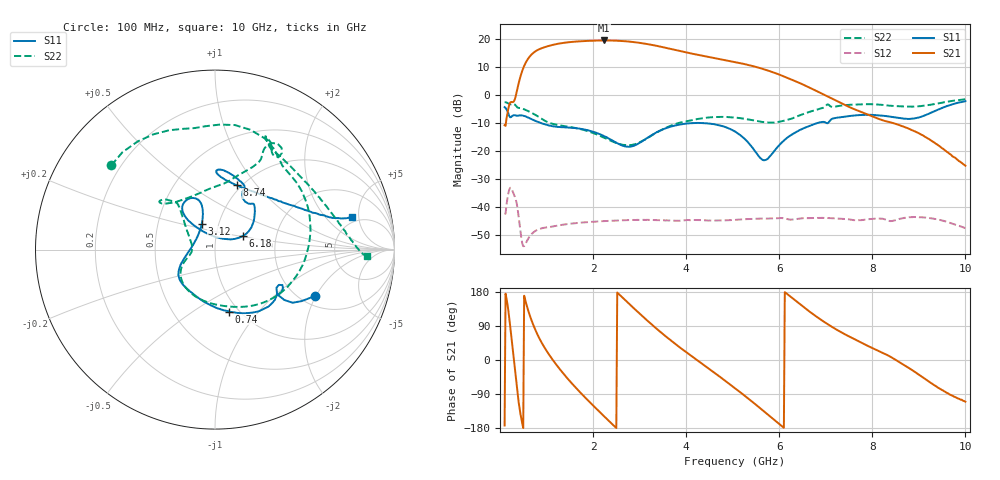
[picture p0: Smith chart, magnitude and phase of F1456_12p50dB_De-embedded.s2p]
! Integrated Device Technology
! Corporate Headquarters
! 6024 Silver Creek Valley Road
! San Jose, CA 95138  USA
! Phone:  1-408-284-8200
! Toll Free:  1-800-223-1366
! Webpage:  http://www.idt.com/
! Timing and RF Division
! 515 Groton Road, Suite 102
! Westford, MA 01886-6024
! Device:  F1456
! Description: 6-bit 0.5 dB Transmit Variable Gain Amplifier
! Frequency:  2100.0 -  2950.00 MHz
! Package:  6x6 mm Thin QFN Plastic Package: 28 pin
! State:  25
! Atten State:  12.5 dB
! Voltage:  +5.00 Volts
! Current:  216.995 mA
! Data:  The device was measured on a the F1455 evaluation board which has
!  individual transmission lines to the RF pins.  Data was collected
!  using a calibrated network analyzer.  The evaluation board was
!  de-embedded using a TRL calibration technique.
!  The reference plane is the edge of the package pin.
!  Pin  1 = CSb
!  Pin  2 = DATA
!  Pin  3 = CLK
!  Pin  4 = RSET
!  Pin  5 = GND
!  Pin  6 = RFIN  = Port 1
!  Pin  7 = GND
!  Pin  8 = NC
!  Pin  9 = NC
!  Pin 10 = NC
!  Pin 11 = NC
!  Pin 12 = NC
!  Pin 13 = NC
!  Pin 14 = /STBY
!  Pin 15 = GND
!  Pin 16 = RFOUT  = Port 2
!  Pin 17 = GND
!  Pin 18 = NC
!  Pin 19 = NC
!  Pin 20 = NC
!  Pin 21 = GND
!  Pin 22 = NC
!  Pin 23 = GND
!  Pin 24 = NC
!  Pin 25 = NC
!  Pin 26 = NC
!  Pin 27 = GND
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# GHz S dB R 50
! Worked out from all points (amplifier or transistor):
!   496 points, 100 MHz to 10 GHz, reference 50 ohm
!   highest |S21| = 19.6 dB at 2.24 GHz (marker M1)
!   |S21| within 3 dB of that: 862.8 MHz to 3.663 GHz (2.8 GHz wide, 124 % of centre)
!   unconditionally stable (mu >= 1): start of sweep to end of sweep
!   at 1.74 GHz: K = 9.13, MAG = 19.9 dB, |S12| = -45.6 dB
!   at 5.06 GHz: K = 17.41, MAG = 12.8 dB, |S12| = -44.6 dB
!   at 10 GHz: K = 241.91, MAG = -15.7 dB, |S12| = -47.5 dB
!   S11 on the Smith chart (normalised r, x): 100 MHz: 2.35, -1.96; 740 MHz: 0.90, -0.71; 3.12 GHz: 0.83, +0.25; 6.18 GHz: 1.35, +0.21; 8.74 GHz: 0.96, +0.80; 10 GHz: 4.31, +4.02
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0.1  -4.26 -25.1  -10.71 -172.9  -42.30 47.0  -2.57 140.9
0.32  -7.15 -32.5  -1.43 -21.4  -36.37 -143.7  -3.36 66.1
0.44  -7.21 -42.4  6.68 -142.0  -48.69 139.6  -4.61 38.7
0.58  -7.79 -59.5  12.43 141.6  -52.16 169.3  -5.48 6.7
0.74  -9.02 -77.2  15.46 85.3  -48.81 137.3  -6.82 -26.4
0.98  -10.48 -100.8  17.31 28.3  -47.35 92.4  -9.27 -68.2
1.2  -11.26 -117.8  18.26 -10.6  -46.78 67.4  -10.51 -96.1
1.5  -11.61 -134.8  19.01 -55.6  -46.00 42.1  -11.35 -124.6
1.76  -12.09 -145.2  19.34 -90.1  -45.57 24.5  -12.24 -141.2
2.24  -14.65 -162.3  19.60 -148.8  -45.04 -2.6  -15.22 -160.7
2.64  -18.09 167.1  19.39 163.9  -44.75 -23.4  -17.76 -176.3
3.12  -15.83 116.9  18.43 109.2  -44.62 -47.5  -15.86 153.3
3.4  -13.01 107.8  17.56 79.0  -44.72 -60.9  -13.07 139.2
3.74  -10.94 107.7  16.31 45.0  -44.91 -75.3  -10.47 130.7
4.1  -10.01 114.5  14.96 11.9  -44.75 -90.4  -9.01 130.9
5.06  -13.07 132.5  11.86 -75.3  -44.60 -132.5  -8.00 139.4
5.64  -23.12 85.9  9.46 -132.2  -44.15 -163.6  -9.57 123.6
6.18  -15.12 26.0  6.15 173.3  -44.37 163.6  -8.77 84.7
6.7  -10.65 41.2  2.33 123.3  -43.92 136.7  -5.70 64.8
8.36  -7.60 87.4  -9.58 10.6  -44.97 66.4  -3.74 62.3
8.74  -8.43 70.8  -11.69 -17.6  -43.80 56.9  -4.06 49.1
10  -2.14 13.4  -25.24 -110.0  -47.55 -24.9  -1.46 -2.6
